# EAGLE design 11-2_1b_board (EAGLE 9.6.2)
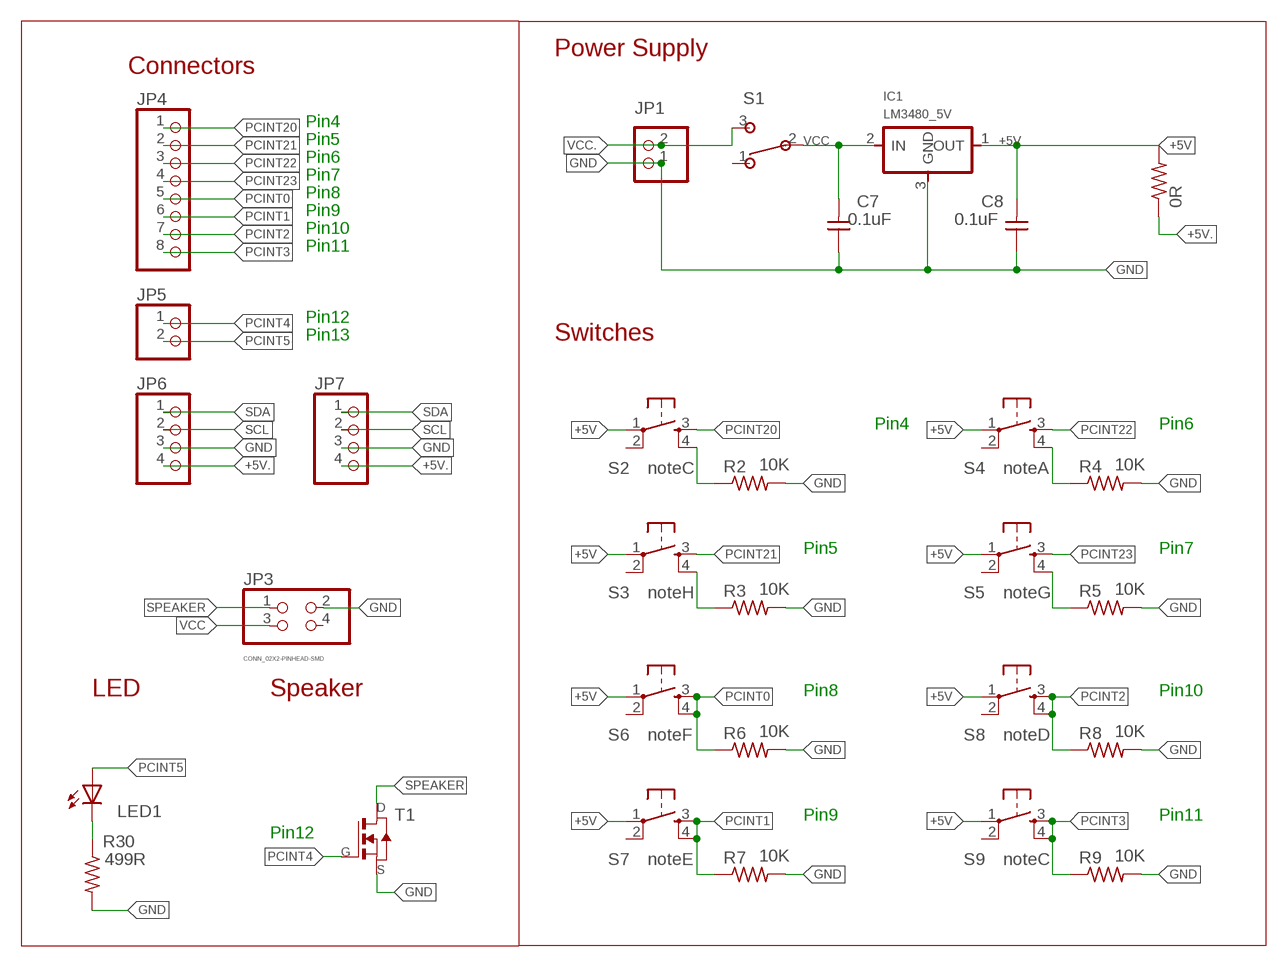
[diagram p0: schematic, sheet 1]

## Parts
C7  0.1uF  CAP_UNPOLARIZEDFAB  [C1206FAB]
C8  0.1uF  CAP_UNPOLARIZEDFAB  [C1206FAB]
IC1  LM3480_5V  VR_REGULATOR-SOT23SOT23  [SOT23]
JP1  PINHD-1X2  [1X02]
JP3  CONN_02X2-PINHEAD-SMD  [2X02SMD]
JP4  PINHD-1X8  [1X08]
JP5  PINHD-1X2  [1X02]
JP6  PINHD-1X4  [1X04]
JP7  PINHD-1X4  [1X04]
LED1  LEDFAB1206  [LED1206FAB]
R2  10K  R1206FAB  [R1206FAB]
R3  10K  R1206FAB  [R1206FAB]
R4  10K  R1206FAB  [R1206FAB]
R5  10K  R1206FAB  [R1206FAB]
R6  10K  R1206FAB  [R1206FAB]
R7  10K  R1206FAB  [R1206FAB]
R8  10K  R1206FAB  [R1206FAB]
R9  10K  R1206FAB  [R1206FAB]
R11  0R  R1206FAB  [R1206FAB]
R30  499R  R1206FAB  [R1206FAB]
S1  SW_SLIDE-SWITCH  [AYZ0102AGRLC]
S2  noteC  SW_SWITCH_TACTILE_6MM6MM_SWITCH  [6MM_SWITCH]
S3  noteH  SW_SWITCH_TACTILE_6MM6MM_SWITCH  [6MM_SWITCH]
S4  noteA  SW_SWITCH_TACTILE_6MM6MM_SWITCH  [6MM_SWITCH]
S5  noteG  SW_SWITCH_TACTILE_6MM6MM_SWITCH  [6MM_SWITCH]
S6  noteF  SW_SWITCH_TACTILE_6MM6MM_SWITCH  [6MM_SWITCH]
S7  noteE  SW_SWITCH_TACTILE_6MM6MM_SWITCH  [6MM_SWITCH]
S8  noteD  SW_SWITCH_TACTILE_6MM6MM_SWITCH  [6MM_SWITCH]
S9  noteC  SW_SWITCH_TACTILE_6MM6MM_SWITCH  [6MM_SWITCH]
T1  MOSFET_NSOT23  [SOT-23]

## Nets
+5V: C8.2 IC1.1(OUT) R11.2 S2.1(P) S3.1(P) S4.1(P) S5.1(P) S6.1(P) S7.1(P) S8.1(P) S9.1(P)
+5V.: JP6.4 JP7.4 R11.1
GND: C7.1 C8.1 IC1.3(GND) JP1.1 JP3.2 JP6.3 JP7.3 R2.2 R3.2 R4.2 R5.2 R6.2 R7.2 R8.2 R9.2 R30.2 T1.2(S)
N$1: LED1.2(C) R30.1
PCINT0: JP4.5 R6.1 S6.3(S) S6.4(S1)
PCINT1: JP4.6 R7.1 S7.3(S) S7.4(S1)
PCINT2: JP4.7 R8.1 S8.3(S) S8.4(S1)
PCINT3: JP4.8 R9.1 S9.3(S) S9.4(S1)
PCINT4: JP5.1 T1.3(G)
PCINT5: JP5.2 LED1.1(A)
PCINT20: JP4.1 R2.1 S2.3(S) S2.4(S1)
PCINT21: JP4.2 S3.3(S)
PCINT21.: R3.1 S3.4(S1)
PCINT22: JP4.3 S4.3(S)
PCINT22.: R4.1 S4.4(S1)
PCINT23: JP4.4 S5.3(S)
PCINT23.: R5.1 S5.4(S1)
SCL: JP6.2 JP7.2
SDA: JP6.1 JP7.1
SPEAKER: JP3.1 T1.1(D)
VCC: C7.2 IC1.2(IN) JP3.3 S1.2
VCC.: JP1.2 S1.3
Unconnected: JP3.4 S1.1 S2.2(P1) S3.2(P1) S4.2(P1) S5.2(P1) S6.2(P1) S7.2(P1) S8.2(P1) S9.2(P1)

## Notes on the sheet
- Power Supply
- Connectors
- Pin4
- Pin5
- Pin6
- Pin7
- Pin8
- Pin9
- Pin10
- Pin11
- Pin12
- Pin13 | Switches
- Pin4 | Pin6
- Pin5 | Pin7
- LED | Speaker | Pin8 | Pin10
- Pin9 | Pin11
- Pin12

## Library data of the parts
C7 C8 = fab:CAP_UNPOLARIZED
IC1 = fab:VR_REGULATOR-SOT23
JP1 JP5 = pinhead:PINHD-1X2: PIN HEADER
JP3 = fab:CONN_02X2-PINHEAD-SMD
JP4 = pinhead:PINHD-1X8: PIN HEADER
JP6 JP7 = pinhead:PINHD-1X4: PIN HEADER
LED1 = fab:LED: LED
R2-R9 R11 R30 = fab:R: Resistor (US Symbol)
S1 = fab:SW_SLIDE-SWITCH: SMD slide-switch AYZ0102AGRLC as found in the fablab inventory. Includes the mounting holes. Made by Zaerc.
S2-S9 = fab:SW_SWITCH_TACTILE_6MM: OMRON SWITCH
T1 = fab:MOSFET_N: MOS FET

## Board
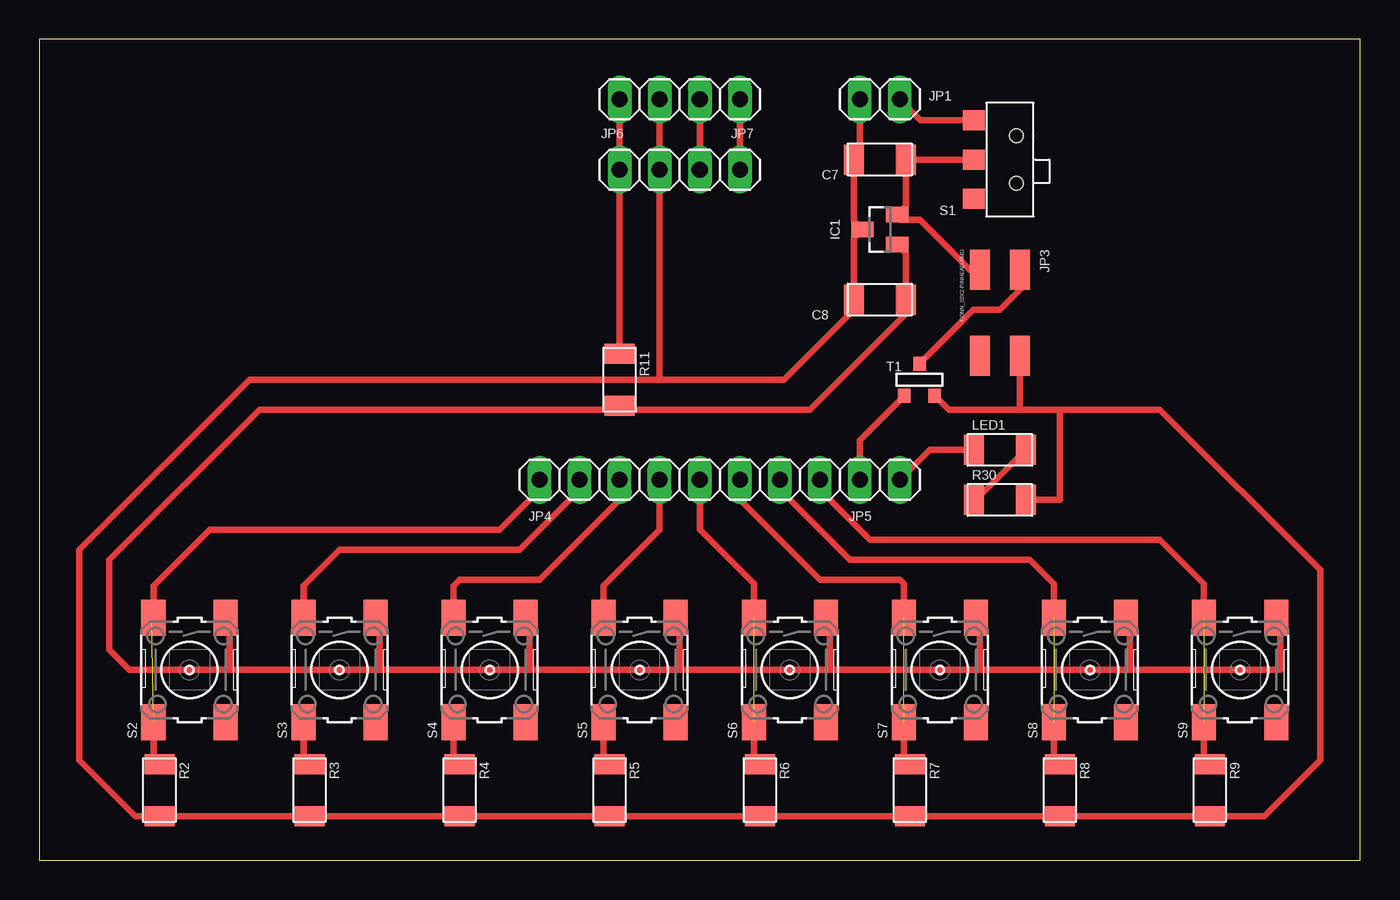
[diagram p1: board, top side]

Size 83.82 x 52.07 mm. Coordinates in mm from the lower left corner, seen from the top.
Outline: 0,0 83.82,0 83.82,52.07 0,52.07 0,0
Copper layers (1*16): Top 0.035mm / dielectric 1.5mm / Bottom 0.035mm
Design rules "default": minimum track width 6mil, minimum drill 0.35mm, track to track 6mil, track to pad 6mil, pad to pad 6mil, via to via 6mil, smd to smd 6mil, copper to edge 40mil, drill to drill 6mil, minimum pad ring 10mil, minimum via ring 8mil, stop-mask expansion 4mil, vias tented up to drill 0mil, thermal gap 10mil
tKeepout: area 18.4,23.5 to 28.6,33.7; area 17.1,31.1 to 19.7,33; area 27.3,31.1 to 29.8,33; area 27.3,26.7 to 29.8,28.6; area 17.1,26.7 to 19.7,28.6

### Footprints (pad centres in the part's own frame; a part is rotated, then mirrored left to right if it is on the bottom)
C1206FAB = smd 1.27 x 1.905: 1 -1.651,0; 2 1.651,0
SOT23 = smd 1 x 1.4: 1 -0.95,-1.1; 2 0.95,-1.1; 3 0,1.1
1X02 = drill 1.016 long: 1 -1.27,0; 2 1.27,0
2X02SMD = smd 2.54 x 1.27: 1 -2.54,1.27; 2 2.92,1.27; 3 -2.54,-1.27; 4 2.92,-1.27
1X08 = drill 1.016 long: 1 -8.89,0; 2 -6.35,0; 3 -3.81,0; 4 -1.27,0; 5 1.27,0; 6 3.81,0; 7 6.35,0; 8 8.89,0
1X04 = drill 1.016 long: 1 -3.81,0; 2 -1.27,0; 3 1.27,0; 4 3.81,0
LED1206FAB = smd 1.27 x 1.905: 1 -1.651,0; 2 1.651,0
R1206FAB = smd 1.27 x 1.905: 1 -1.651,0; 2 1.651,0
AYZ0102AGRLC = smd 1.27 x 1.397: 1 2.5,-2.3; 2 0,-2.3; 3 -2.5,-2.3 | hole 0.85: -1.5,0.4; 1.5,0.4
6MM_SWITCH = smd 2.286 x 1.524: 1 -3.302,2.286; 2 3.302,2.286; 3 -3.302,-2.286; 4 3.302,-2.286
SOT-23 = smd 0.787 x 0.889: 1 0.025,-1.016; 2 -0.94,1.016; 3 0.991,1.016

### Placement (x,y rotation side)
C7  53.34,44.45 0 top
C8  53.34,35.56 0 top
IC1  53.34,40.01 90 top
JP1  53.34,48.26 0 top
JP3  60.96,34.92 270 top
JP4  40.64,24.13 0 top
JP5  53.34,24.13 0 top
JP6  40.64,43.81 180 top
JP7  40.64,48.26 180 top
LED1  60.96,26.04 0 top
R2  7.62,4.45 270 top
R3  17.14,4.45 270 top
R4  26.67,4.45 270 top
R5  36.2,4.45 270 top
R6  45.72,4.45 270 top
R7  55.24,4.45 270 top
R8  64.77,4.45 270 top
R9  74.3,4.45 270 top
R11  36.83,30.48 270 top
R30  60.96,22.86 0 top
S1  61.59,44.45 270 top
S2  9.53,12.06 270 top
S3  19.05,12.06 270 top
S4  28.57,12.06 270 top
S5  38.1,12.06 270 top
S6  47.62,12.06 270 top
S7  57.15,12.06 270 top
S8  66.67,12.06 270 top
S9  76.2,12.06 270 top
T1  55.88,30.48 180 top

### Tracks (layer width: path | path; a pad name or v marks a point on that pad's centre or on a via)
+5V
  Top 0.406: 12.06,12.06 21.59,12.06 | S2.1 12.06,15.11 12.06,12.06 | S3.1 21.59,15.11 21.59,12.06 | 21.59,12.06 31.11,12.06 | S4.1 31.11,15.11 31.11,12.06 | 31.11,12.06 40.64,12.06 | 40.64,12.06 50.16,12.06 | 50.16,12.06 59.69,12.06 | S5.1 40.64,15.11 40.64,12.06 | S6.1 50.16,15.11 50.16,12.06 | S7.1 59.69,15.11 59.69,12.06 | 59.69,12.06 69.22,12.06 | S8.1 69.22,15.11 69.22,12.06 | 69.22,12.06 78.74,12.06 78.74,15.11 S9.1 | IC1.1 54.99,38.5 C8.2 54.99,34.67 48.9,28.57 36.83,28.57 | 12.06,12.06 5.71,12.06 4.45,13.34 4.45,19.05 13.97,28.57 36.83,28.57 | R11.2 36.83,28.57
+5V.
  Top 0.406: JP7.4 JP6.4 R11.1
GND
  Top 0.406: R30.2 64.77,22.86 64.77,28.57 | 39.37,30.48 47.24,30.48 51.69,34.92 C8.1 51.69,39.45 IC1.3 51.69,40.56 C7.1 52.07,44.83 JP1.1 | 39.37,30.48 JP6.3 JP7.3 | 39.37,30.48 13.34,30.48 2.54,19.68 2.54,6.35 6.1,2.79 R2.2 R3.2 R4.2 R5.2 R6.2 R7.2 R8.2 R9.2 77.72,2.79 81.28,6.35 81.28,18.41 71.12,28.57 64.77,28.57 | T1.2 57.71,28.57 62.23,28.57 | 62.23,28.57 64.77,28.57 | JP3.2 62.23,28.57
N$1
  Top 0.406: LED1.2 59.44,22.86 R30.1
PCINT0  (1 unrouted)
  Top 0.406: S6.4 45.34,6.73 46.35,5.71 46.1,5.71 R6.1 | 45.32,15.39 S6.3 45.34,17.53 41.91,20.95 JP4.5
PCINT1  (1 unrouted)
  Top 0.406: S7.4 54.86,6.48 R7.1 | 54.61,15.62 S7.3 54.86,17.53 54.61,17.78 49.53,17.78 44.45,22.86 JP4.6
PCINT2  (1 unrouted)
  Top 0.406: S8.4 64.39,6.48 R8.1 | S8.3 64.39,17.53 62.87,19.05 51.44,19.05 46.99,23.5 JP4.7
PCINT3  (1 unrouted)
  Top 0.406: S9.4 73.91,6.48 R9.1 | S9.3 73.91,17.53 71.12,20.32 52.7,20.32 49.53,23.5 JP4.8
PCINT4
  Top 0.406: JP5.1 52.07,26.64 T1.3
PCINT5
  Top 0.406: JP5.2 56.52,26.04 LED1.1
PCINT20  (1 unrouted)
  Top 0.406: S2.4 7.24,6.48 R2.1 | 7.11,15.24 S2.3 7.24,17.4 10.79,20.95 29.21,20.95 31.75,23.5 JP4.1
PCINT21
  Top 0.406: S3.3 16.76,17.4 19.05,19.68 30.48,19.68 34.29,23.5 JP4.2
PCINT21.
  Top 0.406: S3.4 16.76,6.48 R3.1
PCINT22
  Top 0.406: JP4.3 36.83,22.86 31.75,17.78 26.67,17.78 26.29,17.4 S4.3
PCINT22.
  Top 0.406: S4.4 26.29,6.48 R4.1
PCINT23
  Top 0.406: S5.3 35.81,17.4 39.37,20.95 JP4.4
PCINT23.
  Top 0.406: S5.4 35.81,6.48 R5.1
SCL
  Top 0.406: JP7.2 JP6.2
SDA
  Top 0.406: JP7.1 JP6.1
SPEAKER
  Top 0.406: T1.1 59.28,34.92 60.96,34.92 62.23,36.2 JP3.1
VCC
  Top 0.406: JP3.3 59.05,37.47 55.88,40.64 54.61,40.64 54.44,40.81 IC1.2 54.99,41.51 C7.2 S1.2
VCC.
  Top 0.406: JP1.2 55.92,46.95 S1.3

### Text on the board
tTest: GND | VCC | 5V | GND | SCL | SDA | +5V | GND | P4 | P5 | P6 | P7 | P8 | P9 | P10 | P11 | P12 | P13
Measures: OLED 0,96" / 28,5x28 mm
